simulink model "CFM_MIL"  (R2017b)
settings: Solver=FixedStepDiscrete  StartTime=0.0  StopTime=10.0  FixedStep=0.01  RelTol=1e-3  EnableMultiTasking=on
undefined symbols (not defined in the file): ASWTYPE_FALSE, CFM_CONST0_NUMB, CFM_CONST14_NUMB, CFM_CONST1_NUMB, CFM_CONST6_NUMB, CFM_CONST8_NUMB, Enum_CFMBusBarCell, Enum_CFMNTCTemp
libraries: AIWAYS_Powertrain_BMS_lib x17

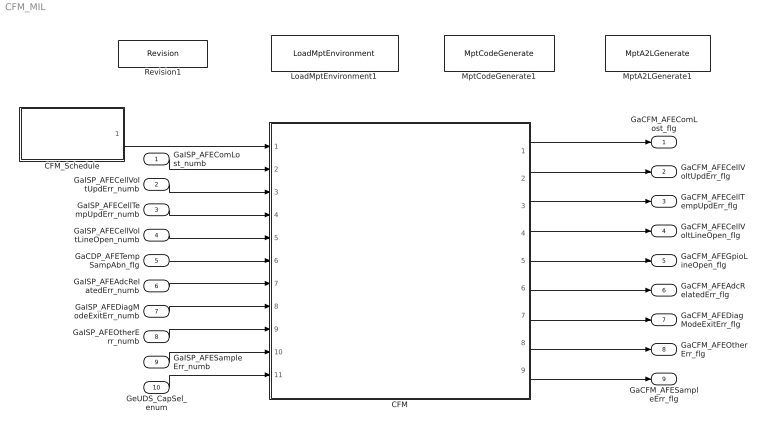
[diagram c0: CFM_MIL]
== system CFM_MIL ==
  GaISP_AFEComLost_numb : Inport
  GaISP_AFECellVoltUpdErr_numb : Inport  Port=2
  GaISP_AFECellTempUpdErr_numb : Inport  Port=3
  GaISP_AFECellVoltLineOpen_numb : Inport  Port=4
  GaCDP_AFETempSampAbn_flg : Inport  Port=5
  GaISP_AFEAdcRelatedErr_numb : Inport  Port=6
  GaISP_AFEDiagModeExitErr_numb : Inport  Port=7
  GaISP_AFEOtherErr_numb : Inport  Port=8
  GaISP_AFESampleErr_numb : Inport  Port=9
  GeUDS_CapSel_enum : Inport  Port=10
  CFM : Subsystem
  CFM_Schedule : Stateflow chart  TreatAsAtomicUnit=on
  LoadMptEnvironment1 : AIWAYS_Powertrain_BMS_lib/Config/LoadMptEnvironment  ProjectName=Comm  SuppierID=NewPlatformUAES
  MptA2LGenerate1 : AIWAYS_Powertrain_BMS_lib/Config/MptA2LGenerate  SystemSampleTime=-1
  MptCodeGenerate1 : AIWAYS_Powertrain_BMS_lib/Config/MptCodeGenerate  SystemSampleTime=-1
  Revision1 : AIWAYS_Powertrain_BMS_lib/Config/Revision  curVersion='M103C102'  newVersion='M103C102'
  GaCFM_AFEComLost_flg : Outport
  GaCFM_AFECellVoltUpdErr_flg : Outport  Port=2
  GaCFM_AFECellTempUpdErr_flg : Outport  Port=3
  GaCFM_AFECellVoltLineOpen_flg : Outport  Port=4
  GaCFM_AFEGpioLineOpen_flg : Outport  Port=5
  GaCFM_AFEAdcRelatedErr_flg : Outport  Port=6
  GaCFM_AFEDiagModeExitErr_flg : Outport  Port=7
  GaCFM_AFEOtherErr_flg : Outport  Port=8
  GaCFM_AFESampleErr_flg : Outport  Port=9
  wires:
  GaISP_AFEComLost_numb/1 -> CFM/2(GaISP_AFEComLost_numb)
  GaISP_AFECellVoltUpdErr_numb/1 -> CFM/3(GaISP_AFECellVoltUpdErr_numb)
  GaISP_AFECellTempUpdErr_numb/1 -> CFM/4(GaISP_AFECellTempUpdErr_numb)
  GaISP_AFECellVoltLineOpen_numb/1 -> CFM/5(GaISP_AFECellVoltLineOpen_numb)
  GaCDP_AFETempSampAbn_flg/1 -> CFM/6(GaCDP_AFETempSampAbn_flg)
  GaISP_AFEAdcRelatedErr_numb/1 -> CFM/7(GaISP_AFEAdcRelatedErr_numb)
  GaISP_AFEDiagModeExitErr_numb/1 -> CFM/8(GaISP_AFEDiagModeExitErr_numb)
  GaISP_AFEOtherErr_numb/1 -> CFM/9(GaISP_AFEOtherErr_numb)
  GaISP_AFESampleErr_numb/1 -> CFM/10(GaISP_AFESampleErr_numb)
  CFM_Schedule/1(CFM_CMCFltMag_20ms()) -> CFM/1(CFM_CMCFltMag_20ms)
  CFM/1(GaCFM_AFEComLost_flg) -> GaCFM_AFEComLost_flg/1
  CFM/2(GaCFM_AFECellVoltUpdErr_flg) -> GaCFM_AFECellVoltUpdErr_flg/1
  CFM/3(GaCFM_AFECellTempUpdErr_flg) -> GaCFM_AFECellTempUpdErr_flg/1
  CFM/4(GaCFM_AFECellVoltLineOpen_flg) -> GaCFM_AFECellVoltLineOpen_flg/1
  CFM/5(GaCFM_AFEGpioLineOpen_flg) -> GaCFM_AFEGpioLineOpen_flg/1
  CFM/6(GaCFM_AFEAdcRelatedErr_flg) -> GaCFM_AFEAdcRelatedErr_flg/1
  CFM/7(GaCFM_AFEDiagModeExitErr_flg) -> GaCFM_AFEDiagModeExitErr_flg/1
  CFM/8(GaCFM_AFEOtherErr_flg) -> GaCFM_AFEOtherErr_flg/1
  CFM/9(GaCFM_AFESampleErr_flg) -> GaCFM_AFESampleErr_flg/1
  GeUDS_CapSel_enum/1 -> CFM/11(GeUDS_CapSel_enum)

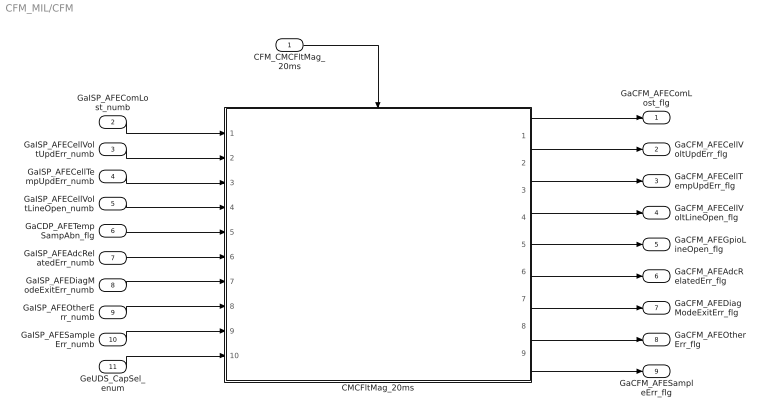
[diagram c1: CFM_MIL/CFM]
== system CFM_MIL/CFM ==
  CFM_CMCFltMag_20ms : Inport
  GaISP_AFEComLost_numb : Inport  Port=2
  GaISP_AFECellVoltUpdErr_numb : Inport  Port=3
  GaISP_AFECellTempUpdErr_numb : Inport  Port=4
  GaISP_AFECellVoltLineOpen_numb : Inport  Port=5
  GaCDP_AFETempSampAbn_flg : Inport  Port=6
  GaISP_AFEAdcRelatedErr_numb : Inport  Port=7
  GaISP_AFEDiagModeExitErr_numb : Inport  Port=8
  GaISP_AFEOtherErr_numb : Inport  Port=9
  GaISP_AFESampleErr_numb : Inport  Port=10
  GeUDS_CapSel_enum : Inport  Port=11
  CMCFltMag_20ms : Subsystem
  GaCFM_AFEComLost_flg : Outport
  GaCFM_AFECellVoltUpdErr_flg : Outport  Port=2
  GaCFM_AFECellTempUpdErr_flg : Outport  Port=3
  GaCFM_AFECellVoltLineOpen_flg : Outport  Port=4
  GaCFM_AFEGpioLineOpen_flg : Outport  Port=5
  GaCFM_AFEAdcRelatedErr_flg : Outport  Port=6
  GaCFM_AFEDiagModeExitErr_flg : Outport  Port=7
  GaCFM_AFEOtherErr_flg : Outport  Port=8
  GaCFM_AFESampleErr_flg : Outport  Port=9
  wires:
  CFM_CMCFltMag_20ms/1 -> CMCFltMag_20ms/Trigger
  GaISP_AFEComLost_numb/1 -> CMCFltMag_20ms/1(GaISP_AFEComLost_numb)
  GaISP_AFECellVoltUpdErr_numb/1 -> CMCFltMag_20ms/2(GaISP_AFECellVoltUpdErr_numb)
  GaISP_AFECellTempUpdErr_numb/1 -> CMCFltMag_20ms/3(GaISP_AFECellTempUpdErr_numb)
  GaISP_AFECellVoltLineOpen_numb/1 -> CMCFltMag_20ms/4(GaISP_AFECellVoltLineOpen_numb)
  GaCDP_AFETempSampAbn_flg/1 -> CMCFltMag_20ms/5(GaCDP_AFETempSampAbn_flg)
  GaISP_AFEAdcRelatedErr_numb/1 -> CMCFltMag_20ms/6(GaISP_AFEAdcRelatedErr_numb)
  GaISP_AFEDiagModeExitErr_numb/1 -> CMCFltMag_20ms/7(GaISP_AFEDiagModeExitErr_numb)
  GaISP_AFEOtherErr_numb/1 -> CMCFltMag_20ms/8(GaISP_AFEOtherErr_numb)
  GaISP_AFESampleErr_numb/1 -> CMCFltMag_20ms/9(GaISP_AFESampleErr_numb)
  CMCFltMag_20ms/1(GaCFM_AFEComLost_flg) -> GaCFM_AFEComLost_flg/1
  CMCFltMag_20ms/2(GaCFM_AFECellVoltUpdErr_flg) -> GaCFM_AFECellVoltUpdErr_flg/1
  CMCFltMag_20ms/3(GaCFM_AFECellTempUpdErr_flg) -> GaCFM_AFECellTempUpdErr_flg/1
  CMCFltMag_20ms/4(GaCFM_AFECellVoltLineOpen_flg) -> GaCFM_AFECellVoltLineOpen_flg/1
  CMCFltMag_20ms/5(GaCFM_AFEGpioLineOpen_flg) -> GaCFM_AFEGpioLineOpen_flg/1
  CMCFltMag_20ms/6(GaCFM_AFEAdcRelatedErr_flg) -> GaCFM_AFEAdcRelatedErr_flg/1
  CMCFltMag_20ms/7(GaCFM_AFEDiagModeExitErr_flg) -> GaCFM_AFEDiagModeExitErr_flg/1
  CMCFltMag_20ms/8(GaCFM_AFEOtherErr_flg) -> GaCFM_AFEOtherErr_flg/1
  CMCFltMag_20ms/9(GaCFM_AFESampleErr_flg) -> GaCFM_AFESampleErr_flg/1
  GeUDS_CapSel_enum/1 -> CMCFltMag_20ms/10(GeUDS_CapSel_enum)

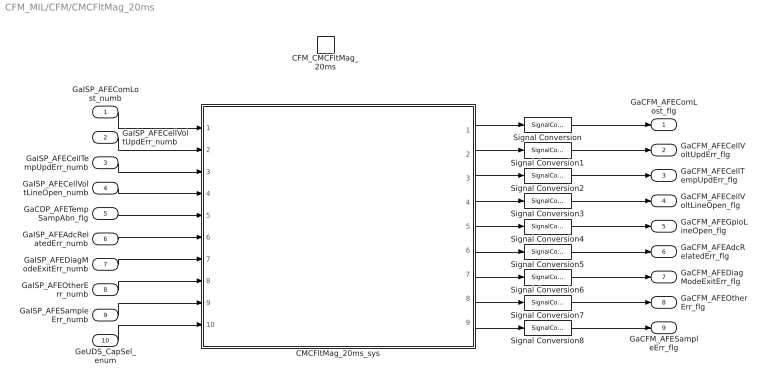
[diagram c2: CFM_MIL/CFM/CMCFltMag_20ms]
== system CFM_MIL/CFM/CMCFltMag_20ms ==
  GaISP_AFEComLost_numb : Inport
  GaISP_AFECellVoltUpdErr_numb : Inport  Port=2
  GaISP_AFECellTempUpdErr_numb : Inport  Port=3
  GaISP_AFECellVoltLineOpen_numb : Inport  Port=4
  GaCDP_AFETempSampAbn_flg : Inport  Port=5
  GaISP_AFEAdcRelatedErr_numb : Inport  Port=6
  GaISP_AFEDiagModeExitErr_numb : Inport  Port=7
  GaISP_AFEOtherErr_numb : Inport  Port=8
  GaISP_AFESampleErr_numb : Inport  Port=9
  GeUDS_CapSel_enum : Inport  Port=10
  CFM_CMCFltMag_20ms : TriggerPort  TriggerType=function-call  VariantControl=(inherit)
  CMCFltMag_20ms_sys : Subsystem
  Signal Conversion{,1..8} (9 alike) : SignalConversion  ConversionOutput=Contiguous copy  OverrideOpt=off
  GaCFM_AFEComLost_flg : Outport
  GaCFM_AFECellVoltUpdErr_flg : Outport  Port=2
  GaCFM_AFECellTempUpdErr_flg : Outport  Port=3
  GaCFM_AFECellVoltLineOpen_flg : Outport  Port=4
  GaCFM_AFEGpioLineOpen_flg : Outport  Port=5
  GaCFM_AFEAdcRelatedErr_flg : Outport  Port=6
  GaCFM_AFEDiagModeExitErr_flg : Outport  Port=7
  GaCFM_AFEOtherErr_flg : Outport  Port=8
  GaCFM_AFESampleErr_flg : Outport  Port=9
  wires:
  GaISP_AFEComLost_numb/1 -> CMCFltMag_20ms_sys/1(GaISP_AFEComLost_numb)
  GaISP_AFECellVoltUpdErr_numb/1 -> CMCFltMag_20ms_sys/2(GaISP_AFECellVoltUpdErr_numb)
  GaISP_AFECellTempUpdErr_numb/1 -> CMCFltMag_20ms_sys/3(GaISP_AFECellTempUpdErr_numb)
  GaISP_AFECellVoltLineOpen_numb/1 -> CMCFltMag_20ms_sys/4(GaISP_AFECellVoltLineOpen_numb)
  GaCDP_AFETempSampAbn_flg/1 -> CMCFltMag_20ms_sys/5(GaCDP_AFETempSampAbn_flg)
  GaISP_AFEAdcRelatedErr_numb/1 -> CMCFltMag_20ms_sys/6(GaISP_AFEAdcRelatedErr_numb)
  GaISP_AFEDiagModeExitErr_numb/1 -> CMCFltMag_20ms_sys/7(GaISP_AFEDiagModeExitErr_numb)
  GaISP_AFEOtherErr_numb/1 -> CMCFltMag_20ms_sys/8(GaISP_AFEOtherErr_numb)
  GaISP_AFESampleErr_numb/1 -> CMCFltMag_20ms_sys/9(GaISP_AFESampleErr_numb)
  CMCFltMag_20ms_sys/1(GaCFM_AFEComLost_flg) -> Signal Conversion/1
  CMCFltMag_20ms_sys/2(GaCFM_AFECellVoltUpdErr_flg) -> Signal Conversion1/1
  CMCFltMag_20ms_sys/3(GaCFM_AFECellTempUpdErr_flg) -> Signal Conversion2/1
  CMCFltMag_20ms_sys/4(GaCFM_AFECellVoltLineOpen_flg) -> Signal Conversion3/1
  CMCFltMag_20ms_sys/5(GaCFM_AFEGpioLineOpen_flg) -> Signal Conversion4/1
  CMCFltMag_20ms_sys/6(GaCFM_AFEAdcRelatedErr_flg) -> Signal Conversion5/1
  CMCFltMag_20ms_sys/7(GaCFM_AFEDiagModeExitErr_flg) -> Signal Conversion6/1
  CMCFltMag_20ms_sys/8(GaCFM_AFEOtherErr_flg) -> Signal Conversion7/1
  CMCFltMag_20ms_sys/9(GaCFM_AFESampleErr_flg) -> Signal Conversion8/1
  Signal Conversion/1 -> GaCFM_AFEComLost_flg/1
  Signal Conversion1/1 -> GaCFM_AFECellVoltUpdErr_flg/1
  Signal Conversion2/1 -> GaCFM_AFECellTempUpdErr_flg/1
  Signal Conversion3/1 -> GaCFM_AFECellVoltLineOpen_flg/1
  Signal Conversion4/1 -> GaCFM_AFEGpioLineOpen_flg/1
  Signal Conversion5/1 -> GaCFM_AFEAdcRelatedErr_flg/1
  Signal Conversion6/1 -> GaCFM_AFEDiagModeExitErr_flg/1
  Signal Conversion7/1 -> GaCFM_AFEOtherErr_flg/1
  Signal Conversion8/1 -> GaCFM_AFESampleErr_flg/1
  GeUDS_CapSel_enum/1 -> CMCFltMag_20ms_sys/10(GeUDS_CapSel_enum)

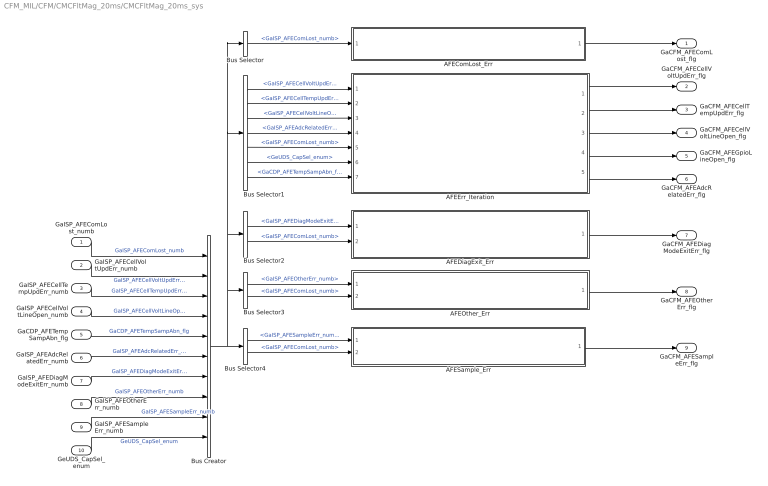
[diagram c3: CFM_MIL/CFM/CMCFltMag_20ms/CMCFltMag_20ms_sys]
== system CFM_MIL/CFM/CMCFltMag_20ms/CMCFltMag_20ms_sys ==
  GaISP_AFEComLost_numb : Inport
  GaISP_AFECellVoltUpdErr_numb : Inport  Port=2
  GaISP_AFECellTempUpdErr_numb : Inport  Port=3
  GaISP_AFECellVoltLineOpen_numb : Inport  Port=4
  GaCDP_AFETempSampAbn_flg : Inport  Port=5
  GaISP_AFEAdcRelatedErr_numb : Inport  Port=6
  GaISP_AFEDiagModeExitErr_numb : Inport  Port=7
  GaISP_AFEOtherErr_numb : Inport  Port=8
  GaISP_AFESampleErr_numb : Inport  Port=9
  GeUDS_CapSel_enum : Inport  Port=10
  AFEComLost_Err : Subsystem
  AFEDiagExit_Err : Subsystem
  AFEErr_Iteration : Subsystem
  AFEOther_Err : Subsystem
  AFESample_Err : Subsystem
  Bus Creator : BusCreator  Inputs=10
  Bus Selector : BusSelector  OutputSignals=GaISP_AFEComLost_numb
  Bus Selector1 : BusSelector  OutputSignals=GaISP_AFECellVoltUpdErr_numb,GaISP_AFECellTempUpdErr_numb,GaISP_AFECellVoltLineOpen_numb,GaISP_AFEAdcRelatedErr_numb,GaISP_AFEComLost_numb,GeUDS_CapSel_enum,GaCDP_AFETempSampAbn_flg
  Bus Selector2 : BusSelector  OutputSignals=GaISP_AFEDiagModeExitErr_numb,GaISP_AFEComLost_numb
  Bus Selector3 : BusSelector  OutputSignals=GaISP_AFEOtherErr_numb,GaISP_AFEComLost_numb
  Bus Selector4 : BusSelector  OutputSignals=GaISP_AFESampleErr_numb,GaISP_AFEComLost_numb
  GaCFM_AFEComLost_flg : Outport
  GaCFM_AFECellVoltUpdErr_flg : Outport  Port=2
  GaCFM_AFECellTempUpdErr_flg : Outport  Port=3
  GaCFM_AFECellVoltLineOpen_flg : Outport  Port=4
  GaCFM_AFEGpioLineOpen_flg : Outport  Port=5
  GaCFM_AFEAdcRelatedErr_flg : Outport  Port=6
  GaCFM_AFEDiagModeExitErr_flg : Outport  Port=7
  GaCFM_AFEOtherErr_flg : Outport  Port=8
  GaCFM_AFESampleErr_flg : Outport  Port=9
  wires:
  AFEComLost_Err/1(GaCFM_AFEComLost_flg) -> GaCFM_AFEComLost_flg/1
  AFEDiagExit_Err/1(GaCFM_AFEDiagModeExitErr_flg) -> GaCFM_AFEDiagModeExitErr_flg/1
  AFEOther_Err/1(GaCFM_AFEOtherErr_flg) -> GaCFM_AFEOtherErr_flg/1
  AFESample_Err/1(GaCFM_AFESampleErr_flg) -> GaCFM_AFESampleErr_flg/1
  AFEErr_Iteration/1(GaCFM_AFECellVoltUpdErr_flg) -> GaCFM_AFECellVoltUpdErr_flg/1
  AFEErr_Iteration/2(GaCFM_AFECellTempUpdErr_flg) -> GaCFM_AFECellTempUpdErr_flg/1
  AFEErr_Iteration/3(GaCFM_AFECellVoltLineOpen_flg) -> GaCFM_AFECellVoltLineOpen_flg/1
  AFEErr_Iteration/4(GaCFM_AFEGpioLineOpen_flg) -> GaCFM_AFEGpioLineOpen_flg/1
  AFEErr_Iteration/5(GaCFM_AFEAdcRelatedErr_flg) -> GaCFM_AFEAdcRelatedErr_flg/1
  GaISP_AFEComLost_numb/1 -> Bus Creator/1  "GaISP_AFEComLost_numb"
  GaISP_AFECellVoltUpdErr_numb/1 -> Bus Creator/2  "GaISP_AFECellVoltUpdErr_numb"
  GaISP_AFECellTempUpdErr_numb/1 -> Bus Creator/3  "GaISP_AFECellTempUpdErr_numb"
  GaISP_AFECellVoltLineOpen_numb/1 -> Bus Creator/4  "GaISP_AFECellVoltLineOpen_numb"
  GaCDP_AFETempSampAbn_flg/1 -> Bus Creator/5  "GaCDP_AFETempSampAbn_flg"
  GaISP_AFEAdcRelatedErr_numb/1 -> Bus Creator/6  "GaISP_AFEAdcRelatedErr_numb"
  GaISP_AFEDiagModeExitErr_numb/1 -> Bus Creator/7  "GaISP_AFEDiagModeExitErr_numb"
  GaISP_AFEOtherErr_numb/1 -> Bus Creator/8  "GaISP_AFEOtherErr_numb"
  GaISP_AFESampleErr_numb/1 -> Bus Creator/9  "GaISP_AFESampleErr_numb"
  Bus Creator/1 -> Bus Selector/1, Bus Selector1/1, Bus Selector2/1, Bus Selector3/1, Bus Selector4/1
  Bus Selector/1 -> AFEComLost_Err/1(GaISP_AFEComLost_numb)  "<GaISP_AFEComLost_numb>"
  Bus Selector2/1 -> AFEDiagExit_Err/1(GaISP_AFEDiagModeExitErr_numb)  "<GaISP_AFEDiagModeExitErr_numb>"
  Bus Selector2/2 -> AFEDiagExit_Err/2(GaISP_AFEComLost_numb)  "<GaISP_AFEComLost_numb>"
  Bus Selector3/1 -> AFEOther_Err/1(GaISP_AFEOtherErr_numb)  "<GaISP_AFEOtherErr_numb>"
  Bus Selector3/2 -> AFEOther_Err/2(GaISP_AFEComLost_numb)  "<GaISP_AFEComLost_numb>"
  Bus Selector4/2 -> AFESample_Err/2(GaISP_AFEComLost_numb)  "<GaISP_AFEComLost_numb>"
  Bus Selector4/1 -> AFESample_Err/1(GaISP_AFESampleErr_numb)  "<GaISP_AFESampleErr_numb>"
  GeUDS_CapSel_enum/1 -> Bus Creator/10  "GeUDS_CapSel_enum"
  Bus Selector1/1 -> AFEErr_Iteration/1(GaISP_AFECellVoltUpdErr_numb)  "<GaISP_AFECellVoltUpdErr_numb>"
  Bus Selector1/2 -> AFEErr_Iteration/2(GaISP_AFECellTempUpdErr_numb)  "<GaISP_AFECellTempUpdErr_numb>"
  Bus Selector1/3 -> AFEErr_Iteration/3(GaISP_AFECellVoltLineOpen_numb)  "<GaISP_AFECellVoltLineOpen_numb>"
  Bus Selector1/4 -> AFEErr_Iteration/4(GaISP_AFEAdcRelatedErr_numb)  "<GaISP_AFEAdcRelatedErr_numb>"
  Bus Selector1/5 -> AFEErr_Iteration/5(GaISP_AFEComLost_numb)  "<GaISP_AFEComLost_numb>"
  Bus Selector1/6 -> AFEErr_Iteration/6(GeUDS_CapSel_enum)  "<GeUDS_CapSel_enum>"
  Bus Selector1/7 -> AFEErr_Iteration/7(GaCDP_AFETempSampAbn_flg)  "<GaCDP_AFETempSampAbn_flg>"

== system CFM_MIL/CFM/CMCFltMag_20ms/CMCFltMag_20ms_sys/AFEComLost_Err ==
  GaISP_AFEComLost_numb : Inport
  CFM_GaCFM_AFEComLost_flg : AIWAYS_Powertrain_BMS_lib/Signals/OverWrite  OverWrite_Value=CaCFM_AFEComLostOvr_flg  OverWrite_flag=CbCFM_AFEComLostOvrSwt_flg
  Constant3 : Constant  Value=CFM_CONST0_NUMB
  Relational Operator2 : RelationalOperator  Operator=~=  OutDataTypeStr=boolean
  GaCFM_AFEComLost_flg : Outport
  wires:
  GaISP_AFEComLost_numb/1 -> Relational Operator2/1
  Constant3/1 -> Relational Operator2/2
  CFM_GaCFM_AFEComLost_flg/1 -> GaCFM_AFEComLost_flg/1  "GaCFM_AFEComLost_flg"
  Relational Operator2/1 -> CFM_GaCFM_AFEComLost_flg/1  "LaCFM_AFEComLost_flg"

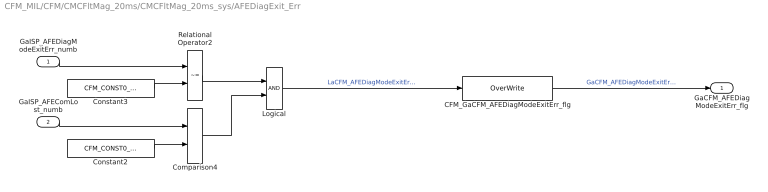
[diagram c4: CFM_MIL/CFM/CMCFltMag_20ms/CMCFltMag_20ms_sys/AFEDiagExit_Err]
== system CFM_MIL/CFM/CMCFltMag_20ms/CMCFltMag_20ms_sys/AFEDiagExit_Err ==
  GaISP_AFEDiagModeExitErr_numb : Inport
  GaISP_AFEComLost_numb : Inport  Port=2
  CFM_GaCFM_AFEDiagModeExitErr_flg : AIWAYS_Powertrain_BMS_lib/Signals/OverWrite  OverWrite_Value=CaCFM_AFEDiagModeExitErrOvr_flg  OverWrite_flag=CbCFM_AFEDiagModeExitErrOvrSwt_flg
  Comparison4 : RelationalOperator  Operator===  OutDataTypeStr=boolean
  Constant2 : Constant  Value=CFM_CONST0_NUMB
  Constant3 : Constant  Value=CFM_CONST0_NUMB
  Logical : Logic  OutDataTypeStr=boolean
  Relational Operator2 : RelationalOperator  Operator=~=  OutDataTypeStr=boolean
  GaCFM_AFEDiagModeExitErr_flg : Outport
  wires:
  Constant3/1 -> Relational Operator2/2
  GaISP_AFEDiagModeExitErr_numb/1 -> Relational Operator2/1
  CFM_GaCFM_AFEDiagModeExitErr_flg/1 -> GaCFM_AFEDiagModeExitErr_flg/1  "GaCFM_AFEDiagModeExitErr_flg"
  Constant2/1 -> Comparison4/2
  GaISP_AFEComLost_numb/1 -> Comparison4/1
  Relational Operator2/1 -> Logical/1
  Comparison4/1 -> Logical/2
  Logical/1 -> CFM_GaCFM_AFEDiagModeExitErr_flg/1  "LaCFM_AFEDiagModeExitErr_flg"

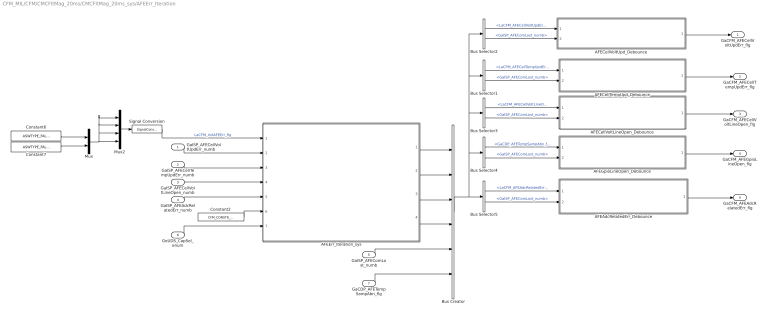
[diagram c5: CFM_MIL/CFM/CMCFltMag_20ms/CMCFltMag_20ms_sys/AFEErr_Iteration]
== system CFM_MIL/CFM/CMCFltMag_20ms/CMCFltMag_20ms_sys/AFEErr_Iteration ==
  GaISP_AFECellVoltUpdErr_numb : Inport
  GaISP_AFECellTempUpdErr_numb : Inport  Port=2
  GaISP_AFECellVoltLineOpen_numb : Inport  Port=3
  GaISP_AFEAdcRelatedErr_numb : Inport  Port=4
  GaISP_AFEComLost_numb : Inport  Port=5
  GeUDS_CapSel_enum : Inport  Port=6
  GaCDP_AFETempSampAbn_flg : Inport  Port=7
  AFEAdcRelatedErr_Debounce : Subsystem
  AFECellTempUpd_Debounce : Subsystem
  AFECellVoltLineOpen_Debounce : Subsystem
  AFECellVoltUpd_Debounce : Subsystem
  AFEErr_Iteration_sys : Subsystem
  AFEGpioLineOpen_Debounce : Subsystem
  Bus Creator : BusCreator  Inputs=6
  Bus Selector1 : BusSelector  OutputSignals=LaCFM_AFECellTempUpdErr_flg,GaISP_AFEComLost_numb
  Bus Selector2 : BusSelector  OutputSignals=LaCFM_AFECellVoltUpdErr_flg,GaISP_AFEComLost_numb
  Bus Selector3 : BusSelector  OutputSignals=LaCFM_AFECellVoltLineOpen_flg,GaISP_AFEComLost_numb
  Bus Selector4 : BusSelector  OutputSignals=GaCDP_AFETempSampAbn_flg,GaISP_AFEComLost_numb
  Bus Selector5 : BusSelector  OutputSignals=LaCFM_AFEAdcRelatedErr_flg,GaISP_AFEComLost_numb
  Constant2 : Constant  Value=CFM_CONST8_NUMB
  Constant6 : Constant  Value=ASWTYPE_FALSE
  Constant7 : Constant  Value=ASWTYPE_FALSE
  Mux : Mux  Inputs=2
  Mux2 : Mux
  Signal Conversion : SignalConversion  ConversionOutput=Contiguous copy  OverrideOpt=off
  GaCFM_AFECellVoltUpdErr_flg : Outport
  GaCFM_AFECellTempUpdErr_flg : Outport  Port=2
  GaCFM_AFECellVoltLineOpen_flg : Outport  Port=3
  GaCFM_AFEGpioLineOpen_flg : Outport  Port=4
  GaCFM_AFEAdcRelatedErr_flg : Outport  Port=5
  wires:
  GaISP_AFECellTempUpdErr_numb/1 -> AFEErr_Iteration_sys/3(GaISP_AFECellTempUpdErr_numb)
  Signal Conversion/1 -> AFEErr_Iteration_sys/1(LaCFM_InitAFEErr_flg)  "LaCFM_InitAFEErr_flg"
  GaISP_AFECellVoltLineOpen_numb/1 -> AFEErr_Iteration_sys/4(GaISP_AFECellVoltLineOpen_numb)
  Constant2/1 -> AFEErr_Iteration_sys/6(CFM_CONST8_NUMB)
  GaISP_AFECellVoltUpdErr_numb/1 -> AFEErr_Iteration_sys/2(GaISP_AFECellVoltUpdErr_numb)
  GaISP_AFEAdcRelatedErr_numb/1 -> AFEErr_Iteration_sys/5(GaISP_AFEAdcRelatedErr_numb)
  Constant6/1 -> Mux/1
  Mux2/1 -> Signal Conversion/1
  Mux/1 -> Mux2/1, Mux2/2, Mux2/3, Mux2/4
  Constant7/1 -> Mux/2
  AFECellVoltUpd_Debounce/1(GaCFM_AFECellVoltUpdErr_flg) -> GaCFM_AFECellVoltUpdErr_flg/1
  AFECellTempUpd_Debounce/1(GaCFM_AFECellTempUpdErr_flg) -> GaCFM_AFECellTempUpdErr_flg/1
  AFECellVoltLineOpen_Debounce/1(GaCFM_AFECellVoltLineOpen_flg) -> GaCFM_AFECellVoltLineOpen_flg/1
  AFEGpioLineOpen_Debounce/1(GaCFM_AFEGpioLineOpen_flg) -> GaCFM_AFEGpioLineOpen_flg/1
  AFEAdcRelatedErr_Debounce/1(GaCFM_AFEAdcRelatedErr_flg) -> GaCFM_AFEAdcRelatedErr_flg/1
  AFEErr_Iteration_sys/1(LaCFM_AFECellVoltUpdErr_flg) -> Bus Creator/1
  AFEErr_Iteration_sys/2(LaCFM_AFECellTempUpdErr_flg) -> Bus Creator/2
  AFEErr_Iteration_sys/3(LaCFM_AFECellVoltLineOpen_flg) -> Bus Creator/3
  AFEErr_Iteration_sys/4(LaCFM_AFEAdcRelatedErr_flg) -> Bus Creator/4
  GaISP_AFEComLost_numb/1 -> Bus Creator/5
  Bus Creator/1 -> Bus Selector1/1, Bus Selector2/1, Bus Selector3/1, Bus Selector4/1, Bus Selector5/1
  Bus Selector2/1 -> AFECellVoltUpd_Debounce/1(LaCFM_AFECellVoltUpdErr_flg)  "<LaCFM_AFECellVoltUpdErr_flg>"
  Bus Selector2/2 -> AFECellVoltUpd_Debounce/2(GaISP_AFEComLost_numb)  "<GaISP_AFEComLost_numb>"
  Bus Selector1/1 -> AFECellTempUpd_Debounce/1(LaCFM_AFECellTempUpdErr_flg)  "<LaCFM_AFECellTempUpdErr_flg>"
  Bus Selector1/2 -> AFECellTempUpd_Debounce/2(GaISP_AFEComLost_numb)  "<GaISP_AFEComLost_numb>"
  Bus Selector3/1 -> AFECellVoltLineOpen_Debounce/1(LaCFM_AFECellVoltLineOpen_flg)  "<LaCFM_AFECellVoltLineOpen_flg>"
  Bus Selector3/2 -> AFECellVoltLineOpen_Debounce/2(GaISP_AFEComLost_numb)  "<GaISP_AFEComLost_numb>"
  Bus Selector4/1 -> AFEGpioLineOpen_Debounce/1(GaCDP_AFETempSampAbn_flg)  "<GaCDP_AFETempSampAbn_flg>"
  Bus Selector4/2 -> AFEGpioLineOpen_Debounce/2(GaISP_AFEComLost_numb)  "<GaISP_AFEComLost_numb>"
  Bus Selector5/1 -> AFEAdcRelatedErr_Debounce/1(LaCFM_AFEAdcRelatedErr_flg)  "<LaCFM_AFEAdcRelatedErr_flg>"
  Bus Selector5/2 -> AFEAdcRelatedErr_Debounce/2(GaISP_AFEComLost_numb)  "<GaISP_AFEComLost_numb>"
  GeUDS_CapSel_enum/1 -> AFEErr_Iteration_sys/7(GeUDS_CapSel_enum)
  GaCDP_AFETempSampAbn_flg/1 -> Bus Creator/6

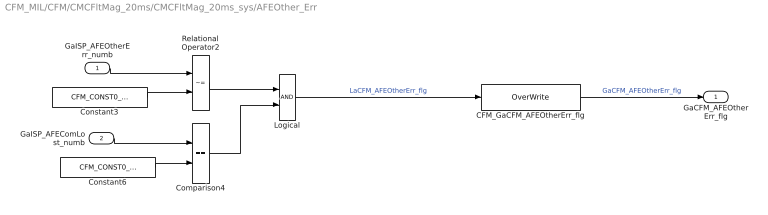
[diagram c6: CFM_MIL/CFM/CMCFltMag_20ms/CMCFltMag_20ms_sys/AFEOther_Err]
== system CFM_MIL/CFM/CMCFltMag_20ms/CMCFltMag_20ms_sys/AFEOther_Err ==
  GaISP_AFEOtherErr_numb : Inport
  GaISP_AFEComLost_numb : Inport  Port=2
  CFM_GaCFM_AFEOtherErr_flg : AIWAYS_Powertrain_BMS_lib/Signals/OverWrite  OverWrite_Value=CaCFM_AFEOtherErrOvr_flg  OverWrite_flag=CbCFM_AFEOtherErrOvrSwt_flg
  Comparison4 : RelationalOperator  Operator===  OutDataTypeStr=boolean
  Constant3 : Constant  Value=CFM_CONST0_NUMB
  Constant6 : Constant  Value=CFM_CONST0_NUMB
  Logical : Logic  OutDataTypeStr=boolean
  Relational Operator2 : RelationalOperator  Operator=~=  OutDataTypeStr=boolean
  GaCFM_AFEOtherErr_flg : Outport
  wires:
  GaISP_AFEOtherErr_numb/1 -> Relational Operator2/1
  Constant3/1 -> Relational Operator2/2
  CFM_GaCFM_AFEOtherErr_flg/1 -> GaCFM_AFEOtherErr_flg/1  "GaCFM_AFEOtherErr_flg"
  Relational Operator2/1 -> Logical/1
  Constant6/1 -> Comparison4/2
  GaISP_AFEComLost_numb/1 -> Comparison4/1
  Comparison4/1 -> Logical/2
  Logical/1 -> CFM_GaCFM_AFEOtherErr_flg/1  "LaCFM_AFEOtherErr_flg"

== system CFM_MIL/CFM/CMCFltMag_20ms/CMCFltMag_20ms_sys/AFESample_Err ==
  GaISP_AFESampleErr_numb : Inport
  GaISP_AFEComLost_numb : Inport  Port=2
  CFM_GaCFM_AFESampleErr_flg : AIWAYS_Powertrain_BMS_lib/Signals/OverWrite  OverWrite_Value=CaCFM_AFESampleErrOvr_flg  OverWrite_flag=CbCFM_AFESampleErrOvrSwt_flg
  Constant2 : Constant  Value=CFM_CONST0_NUMB
  Constant3 : Constant  Value=CFM_CONST0_NUMB
  Logical : Logic  OutDataTypeStr=boolean
  Relational Operator1 : RelationalOperator  Operator===  OutDataTypeStr=boolean
  Relational Operator2 : RelationalOperator  Operator=~=  OutDataTypeStr=boolean
  GaCFM_AFESampleErr_flg : Outport
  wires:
  GaISP_AFESampleErr_numb/1 -> Relational Operator2/1
  Constant3/1 -> Relational Operator2/2
  CFM_GaCFM_AFESampleErr_flg/1 -> GaCFM_AFESampleErr_flg/1  "GaCFM_AFESampleErr_flg"
  Logical/1 -> CFM_GaCFM_AFESampleErr_flg/1  "LaCFM_AFESampleErr_flg"
  Constant2/1 -> Relational Operator1/2
  GaISP_AFEComLost_numb/1 -> Relational Operator1/1
  Relational Operator2/1 -> Logical/1
  Relational Operator1/1 -> Logical/2

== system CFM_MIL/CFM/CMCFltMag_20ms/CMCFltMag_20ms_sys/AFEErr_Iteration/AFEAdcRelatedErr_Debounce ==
  LaCFM_AFEAdcRelatedErr_flg : Inport
  GaISP_AFEComLost_numb : Inport  Port=2
  CFM_GaCFM_AFEAdcRelatedErr_flg : AIWAYS_Powertrain_BMS_lib/Signals/OverWrite  OverWrite_Value=CaCFM_AFEAdcRelatedErrOvr_flg  OverWrite_flag=CbCFM_AFEAdcRelatedErrOvrSwt_flg
  Comparison4 : RelationalOperator  Operator===  OutDataTypeStr=boolean
  Constant3 : Constant  Value=CFM_CONST0_NUMB
  Logical : Logic  OutDataTypeStr=boolean
  GaCFM_AFEAdcRelatedErr_flg : Outport
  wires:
  LaCFM_AFEAdcRelatedErr_flg/1 -> Logical/1
  CFM_GaCFM_AFEAdcRelatedErr_flg/1 -> GaCFM_AFEAdcRelatedErr_flg/1  "GaCFM_AFEAdcRelatedErr_flg"
  Logical/1 -> CFM_GaCFM_AFEAdcRelatedErr_flg/1
  GaISP_AFEComLost_numb/1 -> Comparison4/1
  Comparison4/1 -> Logical/2
  Constant3/1 -> Comparison4/2

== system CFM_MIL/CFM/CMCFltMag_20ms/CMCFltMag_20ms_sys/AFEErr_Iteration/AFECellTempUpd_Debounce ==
  LaCFM_AFECellTempUpdErr_flg : Inport
  GaISP_AFEComLost_numb : Inport  Port=2
  CFM_GaCFM_AFECellTempUpdErr_flg : AIWAYS_Powertrain_BMS_lib/Signals/OverWrite  OverWrite_Value=CaCFM_AFECellTempUpdErrOvr_flg  OverWrite_flag=CbCFM_AFECellTempUpdErrOvrSwt_flg
  Comparison4 : RelationalOperator  Operator===  OutDataTypeStr=boolean
  Constant3 : Constant  Value=CFM_CONST0_NUMB
  Logical : Logic  OutDataTypeStr=boolean
  GaCFM_AFECellTempUpdErr_flg : Outport
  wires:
  CFM_GaCFM_AFECellTempUpdErr_flg/1 -> GaCFM_AFECellTempUpdErr_flg/1  "GaCFM_AFECellTempUpdErr_flg"
  Logical/1 -> CFM_GaCFM_AFECellTempUpdErr_flg/1
  GaISP_AFEComLost_numb/1 -> Comparison4/1
  Comparison4/1 -> Logical/2
  LaCFM_AFECellTempUpdErr_flg/1 -> Logical/1
  Constant3/1 -> Comparison4/2

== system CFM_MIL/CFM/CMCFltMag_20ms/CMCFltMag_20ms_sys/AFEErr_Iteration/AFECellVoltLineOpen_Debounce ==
  LaCFM_AFECellVoltLineOpen_flg : Inport
  GaISP_AFEComLost_numb : Inport  Port=2
  CFM_GaCFM_AFECellVoltLineOpen_flg : AIWAYS_Powertrain_BMS_lib/Signals/OverWrite  OverWrite_Value=CaCFM_AFECellVoltLineOpenOvr_flg  OverWrite_flag=CbCFM_AFECellVoltLineOpenOvrSwt_flg
  Comparison4 : RelationalOperator  Operator===  OutDataTypeStr=boolean
  Constant2 : Constant  Value=CFM_CONST0_NUMB
  Logical : Logic  OutDataTypeStr=boolean
  GaCFM_AFECellVoltLineOpen_flg : Outport
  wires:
  LaCFM_AFECellVoltLineOpen_flg/1 -> Logical/1
  CFM_GaCFM_AFECellVoltLineOpen_flg/1 -> GaCFM_AFECellVoltLineOpen_flg/1  "GaCFM_AFECellVoltLineOpen_flg"
  Logical/1 -> CFM_GaCFM_AFECellVoltLineOpen_flg/1
  GaISP_AFEComLost_numb/1 -> Comparison4/1
  Comparison4/1 -> Logical/2
  Constant2/1 -> Comparison4/2

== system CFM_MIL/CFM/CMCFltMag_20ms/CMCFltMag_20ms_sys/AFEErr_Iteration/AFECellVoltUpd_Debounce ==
  LaCFM_AFECellVoltUpdErr_flg : Inport
  GaISP_AFEComLost_numb : Inport  Port=2
  CFM_GaCFM_AFECellVoltUpdErr_flg : AIWAYS_Powertrain_BMS_lib/Signals/OverWrite  OverWrite_Value=CaCFM_AFECellVoltUpdErrOvr_flg  OverWrite_flag=CbCFM_AFECellVoltUpdErrOvrSwt_flg
  Comparison4 : RelationalOperator  Operator===  OutDataTypeStr=boolean
  Constant3 : Constant  Value=CFM_CONST0_NUMB
  Logical : Logic  OutDataTypeStr=boolean
  GaCFM_AFECellVoltUpdErr_flg : Outport
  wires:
  Logical/1 -> CFM_GaCFM_AFECellVoltUpdErr_flg/1
  CFM_GaCFM_AFECellVoltUpdErr_flg/1 -> GaCFM_AFECellVoltUpdErr_flg/1  "GaCFM_AFECellVoltUpdErr_flg"
  Constant3/1 -> Comparison4/2
  GaISP_AFEComLost_numb/1 -> Comparison4/1
  Comparison4/1 -> Logical/2
  LaCFM_AFECellVoltUpdErr_flg/1 -> Logical/1

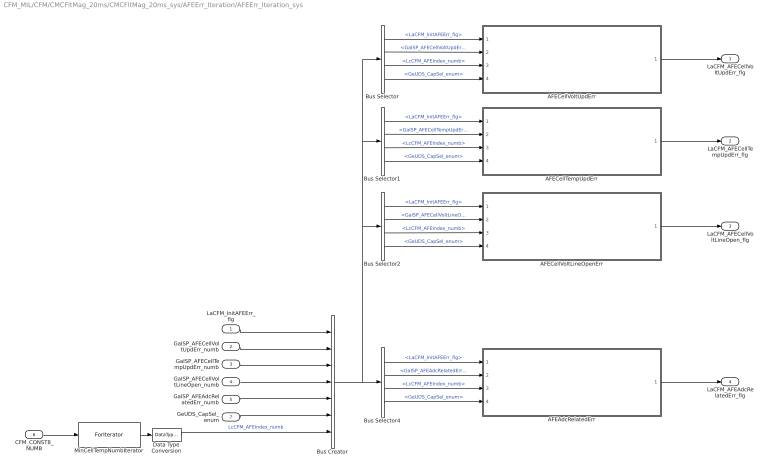
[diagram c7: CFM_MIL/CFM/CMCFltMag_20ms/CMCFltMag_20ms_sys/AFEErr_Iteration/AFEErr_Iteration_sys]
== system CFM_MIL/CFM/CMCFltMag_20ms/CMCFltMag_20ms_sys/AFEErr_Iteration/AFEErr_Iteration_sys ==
  LaCFM_InitAFEErr_flg : Inport
  GaISP_AFECellVoltUpdErr_numb : Inport  Port=2
  GaISP_AFECellTempUpdErr_numb : Inport  Port=3
  GaISP_AFECellVoltLineOpen_numb : Inport  Port=4
  GaISP_AFEAdcRelatedErr_numb : Inport  Port=5
  CFM_CONST8_NUMB : Inport  Port=6
  GeUDS_CapSel_enum : Inport  Port=7
  AFEAdcRelatedErr : Subsystem
  AFECellTempUpdErr : Subsystem
  AFECellVoltLineOpenErr : Subsystem
  AFECellVoltUpdErr : Subsystem
  Bus Creator : BusCreator  Inputs=7
  Bus Selector : BusSelector  OutputSignals=LaCFM_InitAFEErr_flg,GaISP_AFECellVoltUpdErr_numb,LcCFM_AFEIndex_numb,GeUDS_CapSel_enum
  Bus Selector1 : BusSelector  OutputSignals=LaCFM_InitAFEErr_flg,GaISP_AFECellTempUpdErr_numb,LcCFM_AFEIndex_numb,GeUDS_CapSel_enum
  Bus Selector2 : BusSelector  OutputSignals=LaCFM_InitAFEErr_flg,GaISP_AFECellVoltLineOpen_numb,LcCFM_AFEIndex_numb,GeUDS_CapSel_enum
  Bus Selector4 : BusSelector  OutputSignals=LaCFM_InitAFEErr_flg,GaISP_AFEAdcRelatedErr_numb,LcCFM_AFEIndex_numb,GeUDS_CapSel_enum
  Data Type Conversion : DataTypeConversion  OutDataTypeStr=uint8
  MinCellTempNumbIterator : ForIterator  ResetStates=reset  IterationSource=external  IterationVariableDataType=int8
  LaCFM_AFECellVoltUpdErr_flg : Outport
  LaCFM_AFECellTempUpdErr_flg : Outport  Port=2
  LaCFM_AFECellVoltLineOpen_flg : Outport  Port=3
  LaCFM_AFEAdcRelatedErr_flg : Outport  Port=4
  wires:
  MinCellTempNumbIterator/1 -> Data Type Conversion/1
  CFM_CONST8_NUMB/1 -> MinCellTempNumbIterator/1
  LaCFM_InitAFEErr_flg/1 -> Bus Creator/1
  GaISP_AFECellVoltUpdErr_numb/1 -> Bus Creator/2
  Data Type Conversion/1 -> Bus Creator/7  "LcCFM_AFEIndex_numb"
  Bus Creator/1 -> Bus Selector/1, Bus Selector1/1, Bus Selector2/1, Bus Selector4/1
  Bus Selector/1 -> AFECellVoltUpdErr/1(LaCFM_InitAFEErr_flg)  "<LaCFM_InitAFEErr_flg>"
  Bus Selector/2 -> AFECellVoltUpdErr/2(GaISP_AFECellVoltUpdErr_numb)  "<GaISP_AFECellVoltUpdErr_numb>"
  Bus Selector/3 -> AFECellVoltUpdErr/3(LcCFM_AFEIndex_numb)  "<LcCFM_AFEIndex_numb>"
  GaISP_AFECellTempUpdErr_numb/1 -> Bus Creator/3
  GaISP_AFECellVoltLineOpen_numb/1 -> Bus Creator/4
  GaISP_AFEAdcRelatedErr_numb/1 -> Bus Creator/5
  Bus Selector1/1 -> AFECellTempUpdErr/1(LaCFM_InitAFEErr_flg)  "<LaCFM_InitAFEErr_flg>"
  Bus Selector1/2 -> AFECellTempUpdErr/2(GaISP_AFECellTempUpdErr_numb)  "<GaISP_AFECellTempUpdErr_numb>"
  Bus Selector1/3 -> AFECellTempUpdErr/3(LcCFM_AFEIndex_numb)  "<LcCFM_AFEIndex_numb>"
  Bus Selector2/1 -> AFECellVoltLineOpenErr/1(LaCFM_InitAFEErr_flg)  "<LaCFM_InitAFEErr_flg>"
  Bus Selector2/2 -> AFECellVoltLineOpenErr/2(GaISP_AFECellVoltLineOpen_numb)  "<GaISP_AFECellVoltLineOpen_numb>"
  Bus Selector2/3 -> AFECellVoltLineOpenErr/3(LcCFM_AFEIndex_numb)  "<LcCFM_AFEIndex_numb>"
  Bus Selector4/1 -> AFEAdcRelatedErr/1(LaCFM_InitAFEErr_flg)  "<LaCFM_InitAFEErr_flg>"
  Bus Selector4/2 -> AFEAdcRelatedErr/2(GaISP_AFEAdcRelatedErr_numb)  "<GaISP_AFEAdcRelatedErr_numb>"
  Bus Selector4/3 -> AFEAdcRelatedErr/3(LcCFM_AFEIndex_numb)  "<LcCFM_AFEIndex_numb>"
  AFECellVoltLineOpenErr/1(LaCFM_AFECellVoltLineOpen_flg) -> LaCFM_AFECellVoltLineOpen_flg/1
  AFECellTempUpdErr/1(LaCFM_AFECellTempUpdErr_flg) -> LaCFM_AFECellTempUpdErr_flg/1
  AFECellVoltUpdErr/1(LaCFM_AFECellVoltUpdErr_flg) -> LaCFM_AFECellVoltUpdErr_flg/1
  AFEAdcRelatedErr/1(LaCFM_AFEAdcRelatedErr_flg) -> LaCFM_AFEAdcRelatedErr_flg/1
  GeUDS_CapSel_enum/1 -> Bus Creator/6
  Bus Selector/4 -> AFECellVoltUpdErr/4(GeUDS_CapSel_enum)  "<GeUDS_CapSel_enum>"
  Bus Selector1/4 -> AFECellTempUpdErr/4(GeUDS_CapSel_enum)  "<GeUDS_CapSel_enum>"
  Bus Selector2/4 -> AFECellVoltLineOpenErr/4(GeUDS_CapSel_enum)  "<GeUDS_CapSel_enum>"
  Bus Selector4/4 -> AFEAdcRelatedErr/4(GeUDS_CapSel_enum)  "<GeUDS_CapSel_enum>"

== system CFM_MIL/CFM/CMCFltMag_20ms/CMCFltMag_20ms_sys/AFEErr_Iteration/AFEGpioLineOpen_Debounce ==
  GaCDP_AFETempSampAbn_flg : Inport
  GaISP_AFEComLost_numb : Inport  Port=2
  CFM_GaCFM_AFEGpioLineOpen_flg : AIWAYS_Powertrain_BMS_lib/Signals/OverWrite  OverWrite_Value=CaCFM_AFEGpioLineOpenOvr_flg  OverWrite_flag=CbCFM_AFEGpioLineOpenOvrSwt_flg
  Comparison4 : RelationalOperator  Operator===  OutDataTypeStr=boolean
  Constant3 : Constant  Value=CFM_CONST0_NUMB
  Logical : Logic  OutDataTypeStr=boolean
  GaCFM_AFEGpioLineOpen_flg : Outport
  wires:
  Logical/1 -> CFM_GaCFM_AFEGpioLineOpen_flg/1
  CFM_GaCFM_AFEGpioLineOpen_flg/1 -> GaCFM_AFEGpioLineOpen_flg/1  "GaCFM_AFEGpioLineOpen_flg"
  GaISP_AFEComLost_numb/1 -> Comparison4/1
  Comparison4/1 -> Logical/2
  GaCDP_AFETempSampAbn_flg/1 -> Logical/1
  Constant3/1 -> Comparison4/2

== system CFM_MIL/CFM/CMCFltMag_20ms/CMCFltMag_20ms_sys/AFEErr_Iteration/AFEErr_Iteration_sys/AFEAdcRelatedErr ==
  LaCFM_InitAFEErr_flg : Inport
  GaISP_AFEAdcRelatedErr_numb : Inport  Port=2
  LcCFM_AFEIndex_numb : Inport  Port=3
  GeUDS_CapSel_enum : Inport  Port=4
  AFEAdcRelatedErr_sys : Subsystem
  Assignment : Assignment  DiagnosticForDimensions=Warning  IndexOptions=Index vector (port)  Indices=1  OutputSizes=1
  Constant2 : Constant  Value=CFM_CONST14_NUMB
  LaCFM_AFEAdcRelatedErr_flg : Outport
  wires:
  LaCFM_InitAFEErr_flg/1 -> Assignment/1
  GaISP_AFEAdcRelatedErr_numb/1 -> AFEAdcRelatedErr_sys/1(GaISP_AFEAdcRelatedErr_numb)
  LcCFM_AFEIndex_numb/1 -> AFEAdcRelatedErr_sys/2(LcCFM_AFEIndex_numb), Assignment/3
  Constant2/1 -> AFEAdcRelatedErr_sys/3(CFM_CONST14_NUMB)
  AFEAdcRelatedErr_sys/1(LbCFM_AFEAdcRelatedErr_flg) -> Assignment/2
  Assignment/1 -> LaCFM_AFEAdcRelatedErr_flg/1  "LaCFM_AFEAdcRelatedErr_flg"
  GeUDS_CapSel_enum/1 -> AFEAdcRelatedErr_sys/4(GeUDS_CapSel_enum)

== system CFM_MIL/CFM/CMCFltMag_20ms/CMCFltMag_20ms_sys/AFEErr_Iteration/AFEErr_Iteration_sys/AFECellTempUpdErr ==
  LaCFM_InitAFEErr_flg : Inport
  GaISP_AFECellTempUpdErr_numb : Inport  Port=2
  LcCFM_AFEIndex_numb : Inport  Port=3
  GeUDS_CapSel_enum : Inport  Port=4
  AFECellTempUpdErr_sys : Subsystem
  Assignment : Assignment  DiagnosticForDimensions=Warning  IndexOptions=Index vector (port)  Indices=1  OutputSizes=1
  Constant2 : Constant  Value=CFM_CONST6_NUMB
  LaCFM_AFECellTempUpdErr_flg : Outport
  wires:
  Assignment/1 -> LaCFM_AFECellTempUpdErr_flg/1  "LaCFM_AFECellTempUpdErr_flg"
  AFECellTempUpdErr_sys/1(LbCFM_AFETempUpdErr_flg) -> Assignment/2
  Constant2/1 -> AFECellTempUpdErr_sys/3(CFM_CONST6_NUMB)
  LcCFM_AFEIndex_numb/1 -> Assignment/3, AFECellTempUpdErr_sys/2(LcCFM_AFEIndex_numb)
  GaISP_AFECellTempUpdErr_numb/1 -> AFECellTempUpdErr_sys/1(GaISP_AFECellTempUpdErr_numb)
  LaCFM_InitAFEErr_flg/1 -> Assignment/1
  GeUDS_CapSel_enum/1 -> AFECellTempUpdErr_sys/4(GeUDS_CapSel_enum)

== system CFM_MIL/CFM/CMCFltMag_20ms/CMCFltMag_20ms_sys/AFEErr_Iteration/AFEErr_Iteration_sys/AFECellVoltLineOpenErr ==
  LaCFM_InitAFEErr_flg : Inport
  GaISP_AFECellVoltLineOpen_numb : Inport  Port=2
  LcCFM_AFEIndex_numb : Inport  Port=3
  GeUDS_CapSel_enum : Inport  Port=4
  AFECellVoltLineOpenErr_sys : Subsystem
  Assignment : Assignment  DiagnosticForDimensions=Warning  IndexOptions=Index vector (port)  Indices=1  OutputSizes=1
  Constant2 : Constant  Value=CFM_CONST14_NUMB
  LaCFM_AFECellVoltLineOpen_flg : Outport
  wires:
  Assignment/1 -> LaCFM_AFECellVoltLineOpen_flg/1  "LaCFM_AFECellVoltLineOpen_flg"
  AFECellVoltLineOpenErr_sys/1(LbCFM_AFECellVoltLineOpenErr_flg) -> Assignment/2
  Constant2/1 -> AFECellVoltLineOpenErr_sys/3(CFM_CONST14_NUMB)
  LcCFM_AFEIndex_numb/1 -> Assignment/3, AFECellVoltLineOpenErr_sys/2(LcCFM_AFEIndex_numb)
  GaISP_AFECellVoltLineOpen_numb/1 -> AFECellVoltLineOpenErr_sys/1(GaISP_AFECellVoltLineOpen_numb)
  LaCFM_InitAFEErr_flg/1 -> Assignment/1
  GeUDS_CapSel_enum/1 -> AFECellVoltLineOpenErr_sys/4(GeUDS_CapSel_enum)

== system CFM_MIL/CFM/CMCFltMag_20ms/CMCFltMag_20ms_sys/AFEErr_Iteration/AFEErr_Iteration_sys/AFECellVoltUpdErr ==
  LaCFM_InitAFEErr_flg : Inport
  GaISP_AFECellVoltUpdErr_numb : Inport  Port=2
  LcCFM_AFEIndex_numb : Inport  Port=3
  GeUDS_CapSel_enum : Inport  Port=4
  AFECellVoltUpdErr_sys : Subsystem
  Assignment : Assignment  DiagnosticForDimensions=Warning  IndexOptions=Index vector (port)  Indices=1  OutputSizes=1
  Constant2 : Constant  Value=CFM_CONST14_NUMB
  LaCFM_AFECellVoltUpdErr_flg : Outport
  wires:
  LaCFM_InitAFEErr_flg/1 -> Assignment/1
  GaISP_AFECellVoltUpdErr_numb/1 -> AFECellVoltUpdErr_sys/1(GaISP_AFECellVoltUpdErr_numb)
  LcCFM_AFEIndex_numb/1 -> AFECellVoltUpdErr_sys/2(LcCFM_AFEIndex_numb), Assignment/3
  Constant2/1 -> AFECellVoltUpdErr_sys/3(CFM_CONST14_NUMB)
  AFECellVoltUpdErr_sys/1(LbCFM_AFECellVoltUpdErr_flg) -> Assignment/2
  Assignment/1 -> LaCFM_AFECellVoltUpdErr_flg/1  "LaCFM_AFECellVoltUpdErr_flg"
  GeUDS_CapSel_enum/1 -> AFECellVoltUpdErr_sys/4(GeUDS_CapSel_enum)

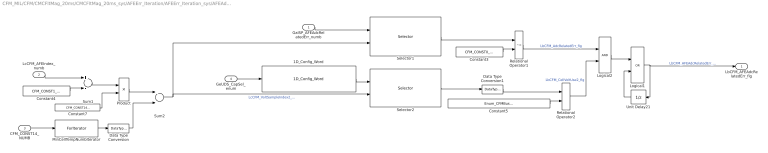
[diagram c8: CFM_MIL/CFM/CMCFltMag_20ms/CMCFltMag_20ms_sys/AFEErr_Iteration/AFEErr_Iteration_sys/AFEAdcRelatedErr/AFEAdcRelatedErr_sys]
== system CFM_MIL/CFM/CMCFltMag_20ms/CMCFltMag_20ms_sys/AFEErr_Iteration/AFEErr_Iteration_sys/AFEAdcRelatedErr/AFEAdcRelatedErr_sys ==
  GaISP_AFEAdcRelatedErr_numb : Inport
  LcCFM_AFEIndex_numb : Inport  Port=2
  CFM_CONST14_NUMB : Inport  Port=3
  GeUDS_CapSel_enum : Inport  Port=4
  1D_Config_Word : AIWAYS_Powertrain_BMS_lib/Signals/1D_Config_Word  Default_CalPar_Name=CaCFM_CATL177BusBarCell_enum  CATL153Ah_CalPar_Name=CaCFM_CATL177BusBarCell_enum  CATL180Ah_CalPar_Name=CaCFM_CATL177BusBarCell_enum  CATL177Ah_CalPar_Name=CaCFM_CATL177BusBarCell_enum  CATL203Ah_CalPar_Name=CaCFM_CATL203BusBarCell_enum  CATL51Ah_CalPar_Name=CaCFM_CATL177BusBarCell_enum  CATL132Ah_CalPar_Name=CaCFM_CATL177BusBarCell_enum  XWD75Ah_CalPar_Name=CaCFM_XWD75BusBarCell_enum  TFE177Ah_CalPar_Name=CaCFM_TFE177BusBarCell_enum  CATLCTP248Ah_CalPar_Name=CaCFM_CATL177BusBarCell_enum
  Constant3 : Constant  Value=CFM_CONST0_NUMB
  Constant4 : Constant  Value=CFM_CONST1_NUMB
  Constant5 : Constant  Value=Enum_CFMBusBarCell.Enum_CFMBusBarCell_Cell
  Constant7 : Constant  Value=CFM_CONST14_NUMB
  Data Type Conversion : DataTypeConversion  OutDataTypeStr=uint16
  Data Type Conversion1 : DataTypeConversion
  Logical1 : Logic  Operator=OR  OutDataTypeStr=boolean
  Logical2 : Logic  OutDataTypeStr=boolean
  MinCellTempNumbIterator : ForIterator  ResetStates=reset  IterationSource=external  IterationVariableDataType=int8
  Product : Product  OutDataTypeStr=Inherit: Inherit via back propagation
  Relational Operator1 : RelationalOperator  Operator=~=  OutDataTypeStr=boolean
  Relational Operator2 : RelationalOperator  Operator===  OutDataTypeStr=boolean
  Selector1 : Selector  IndexOptions=Index vector (port)  Indices=[1 3]  OutputSizes=1
  Selector2 : Selector  IndexOptions=Index vector (port)  Indices=[1 3]  OutputSizes=1
  Sum1 : Sum  Inputs=+-  OutDataTypeStr=Inherit: Inherit via back propagation  RndMeth=Zero
  Sum2 : Sum  OutDataTypeStr=Inherit: Inherit via back propagation  RndMeth=Zero
  Unit Delay21 : UnitDelay  InitialCondition=ASWTYPE_FALSE  SampleTime=-1  StateName=StateName
  LbCFM_AFEAdcRelatedErr_flg : Outport
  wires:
  Relational Operator2/1 -> Logical2/2  "LbCFM_CellVoltUse2_flg"
  Relational Operator1/1 -> Logical2/1  "LbCFM_AdcRelatedErr_flg"
  1D_Config_Word/1 -> Selector2/1
  GaISP_AFEAdcRelatedErr_numb/1 -> Selector1/1
  Constant3/1 -> Relational Operator1/2
  Selector2/1 -> Data Type Conversion1/1
  Constant5/1 -> Relational Operator2/2
  Selector1/1 -> Relational Operator1/1
  CFM_CONST14_NUMB/1 -> MinCellTempNumbIterator/1
  MinCellTempNumbIterator/1 -> Data Type Conversion/1
  Constant4/1 -> Sum1/2
  LcCFM_AFEIndex_numb/1 -> Sum1/1
  Sum1/1 -> Product/1
  Constant7/1 -> Product/2
  Product/1 -> Sum2/1
  Data Type Conversion/1 -> Sum2/2
  Sum2/1 -> Selector2/2, Selector1/2  "LcCFM_VoltSampleIndex2_numb"
  Logical2/1 -> Logical1/1
  Unit Delay21/1 -> Logical1/2
  Logical1/1 -> LbCFM_AFEAdcRelatedErr_flg/1, Unit Delay21/1  "LbCFM_AFEAdcRelatedErr_flg"
  Data Type Conversion1/1 -> Relational Operator2/1
  GeUDS_CapSel_enum/1 -> 1D_Config_Word/1

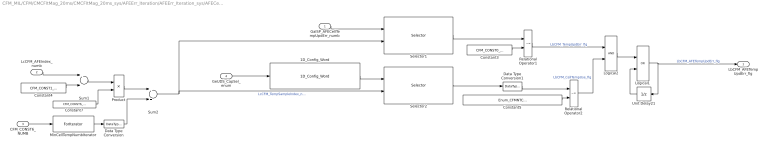
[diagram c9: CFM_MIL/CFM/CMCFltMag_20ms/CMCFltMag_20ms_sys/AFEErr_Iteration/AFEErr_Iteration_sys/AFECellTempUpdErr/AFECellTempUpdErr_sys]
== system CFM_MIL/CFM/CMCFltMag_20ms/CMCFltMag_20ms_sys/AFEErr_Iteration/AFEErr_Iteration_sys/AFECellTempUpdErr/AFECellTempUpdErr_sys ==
  GaISP_AFECellTempUpdErr_numb : Inport
  LcCFM_AFEIndex_numb : Inport  Port=2
  CFM_CONST6_NUMB : Inport  Port=3
  GeUDS_CapSel_enum : Inport  Port=4
  1D_Config_Word : AIWAYS_Powertrain_BMS_lib/Signals/1D_Config_Word  Default_CalPar_Name=CaCFM_CATL177NTCTemp_enum  CATL153Ah_CalPar_Name=CaCFM_CATL177NTCTemp_enum  CATL180Ah_CalPar_Name=CaCFM_CATL177NTCTemp_enum  CATL177Ah_CalPar_Name=CaCFM_CATL177NTCTemp_enum  CATL203Ah_CalPar_Name=CaCFM_CATL203NTCTemp_enum  CATL51Ah_CalPar_Name=CaCFM_CATL177NTCTemp_enum  CATL132Ah_CalPar_Name=CaCFM_CATL177NTCTemp_enum  XWD75Ah_CalPar_Name=CaCFM_XWD75NTCTemp_enum  TFE177Ah_CalPar_Name=CaCFM_TFE177NTCTemp_enum  CATLCTP248Ah_CalPar_Name=CaCFM_CATL177NTCTemp_enum
  Constant3 : Constant  Value=CFM_CONST0_NUMB
  Constant4 : Constant  Value=CFM_CONST1_NUMB
  Constant5 : Constant  Value=Enum_CFMNTCTemp.Enum_CFMNTCTemp_NoUse
  Constant7 : Constant  Value=CFM_CONST6_NUMB
  Data Type Conversion : DataTypeConversion  OutDataTypeStr=uint16
  Data Type Conversion1 : DataTypeConversion
  Logical1 : Logic  Operator=OR  OutDataTypeStr=boolean
  Logical2 : Logic  OutDataTypeStr=boolean
  MinCellTempNumbIterator : ForIterator  ResetStates=reset  IterationSource=external  IterationVariableDataType=int8
  Product : Product  OutDataTypeStr=Inherit: Inherit via back propagation
  Relational Operator1 : RelationalOperator  Operator=~=  OutDataTypeStr=boolean
  Relational Operator2 : RelationalOperator  Operator=~=  OutDataTypeStr=boolean
  Selector1 : Selector  IndexOptions=Index vector (port)  Indices=[1 3]  OutputSizes=1
  Selector2 : Selector  IndexOptions=Index vector (port)  Indices=[1 3]  OutputSizes=1
  Sum1 : Sum  Inputs=+-  OutDataTypeStr=Inherit: Inherit via back propagation  RndMeth=Zero
  Sum2 : Sum  OutDataTypeStr=Inherit: Inherit via back propagation  RndMeth=Zero
  Unit Delay21 : UnitDelay  InitialCondition=ASWTYPE_FALSE  SampleTime=-1  StateName=StateName
  LbCFM_AFETempUpdErr_flg : Outport
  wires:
  Logical1/1 -> Unit Delay21/1, LbCFM_AFETempUpdErr_flg/1  "LbCFM_AFETempUpdErr_flg"
  Unit Delay21/1 -> Logical1/2
  Logical2/1 -> Logical1/1
  Sum2/1 -> Selector2/2, Selector1/2  "LcCFM_TempSampleIndex_numb"
  Data Type Conversion/1 -> Sum2/2
  Product/1 -> Sum2/1
  Constant7/1 -> Product/2
  Sum1/1 -> Product/1
  LcCFM_AFEIndex_numb/1 -> Sum1/1
  Constant4/1 -> Sum1/2
  MinCellTempNumbIterator/1 -> Data Type Conversion/1
  CFM_CONST6_NUMB/1 -> MinCellTempNumbIterator/1
  Selector1/1 -> Relational Operator1/1
  Constant5/1 -> Relational Operator2/2
  Selector2/1 -> Data Type Conversion1/1
  Constant3/1 -> Relational Operator1/2
  GaISP_AFECellTempUpdErr_numb/1 -> Selector1/1
  1D_Config_Word/1 -> Selector2/1
  Relational Operator1/1 -> Logical2/1  "LbCFM_TempUpdErr_flg"
  Relational Operator2/1 -> Logical2/2  "LbCFM_CellTempUse_flg"
  Data Type Conversion1/1 -> Relational Operator2/1
  GeUDS_CapSel_enum/1 -> 1D_Config_Word/1

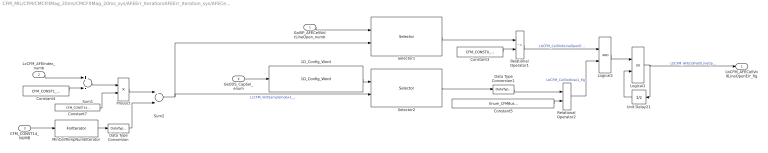
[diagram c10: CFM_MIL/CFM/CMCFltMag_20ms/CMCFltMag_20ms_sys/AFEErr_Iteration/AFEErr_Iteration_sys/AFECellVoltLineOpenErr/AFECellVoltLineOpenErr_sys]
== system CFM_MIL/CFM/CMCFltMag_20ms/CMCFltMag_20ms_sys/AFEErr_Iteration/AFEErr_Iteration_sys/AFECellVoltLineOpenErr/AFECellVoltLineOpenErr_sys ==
  GaISP_AFECellVoltLineOpen_numb : Inport
  LcCFM_AFEIndex_numb : Inport  Port=2
  CFM_CONST14_NUMB : Inport  Port=3
  GeUDS_CapSel_enum : Inport  Port=4
  1D_Config_Word : AIWAYS_Powertrain_BMS_lib/Signals/1D_Config_Word  Default_CalPar_Name=CaCFM_CATL177BusBarCell_enum  CATL153Ah_CalPar_Name=CaCFM_CATL177BusBarCell_enum  CATL180Ah_CalPar_Name=CaCFM_CATL177BusBarCell_enum  CATL177Ah_CalPar_Name=CaCFM_CATL177BusBarCell_enum  CATL203Ah_CalPar_Name=CaCFM_CATL203BusBarCell_enum  CATL51Ah_CalPar_Name=CaCFM_CATL177BusBarCell_enum  CATL132Ah_CalPar_Name=CaCFM_CATL177BusBarCell_enum  XWD75Ah_CalPar_Name=CaCFM_XWD75BusBarCell_enum  TFE177Ah_CalPar_Name=CaCFM_TFE177BusBarCell_enum  CATLCTP248Ah_CalPar_Name=CaCFM_CATL177BusBarCell_enum
  Constant3 : Constant  Value=CFM_CONST0_NUMB
  Constant4 : Constant  Value=CFM_CONST1_NUMB
  Constant5 : Constant  Value=Enum_CFMBusBarCell.Enum_CFMBusBarCell_Cell
  Constant7 : Constant  Value=CFM_CONST14_NUMB
  Data Type Conversion : DataTypeConversion  OutDataTypeStr=uint16
  Data Type Conversion1 : DataTypeConversion
  Logical1 : Logic  Operator=OR  OutDataTypeStr=boolean
  Logical2 : Logic  OutDataTypeStr=boolean
  MinCellTempNumbIterator : ForIterator  ResetStates=reset  IterationSource=external  IterationVariableDataType=int8
  Product : Product  OutDataTypeStr=Inherit: Inherit via back propagation
  Relational Operator1 : RelationalOperator  Operator=~=  OutDataTypeStr=boolean
  Relational Operator2 : RelationalOperator  Operator===  OutDataTypeStr=boolean
  Selector1 : Selector  IndexOptions=Index vector (port)  Indices=[1 3]  OutputSizes=1
  Selector2 : Selector  IndexOptions=Index vector (port)  Indices=[1 3]  OutputSizes=1
  Sum1 : Sum  Inputs=+-  OutDataTypeStr=Inherit: Inherit via back propagation  RndMeth=Zero
  Sum2 : Sum  OutDataTypeStr=Inherit: Inherit via back propagation  RndMeth=Zero
  Unit Delay21 : UnitDelay  InitialCondition=ASWTYPE_FALSE  SampleTime=-1  StateName=StateName
  LbCFM_AFECellVoltLineOpenErr_flg : Outport
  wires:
  Logical1/1 -> Unit Delay21/1, LbCFM_AFECellVoltLineOpenErr_flg/1  "LbCFM_AFECellVoltLineOpenErr_flg"
  Unit Delay21/1 -> Logical1/2
  Logical2/1 -> Logical1/1
  Sum2/1 -> Selector2/2, Selector1/2  "LcCFM_VoltSampleIndex1_numb"
  Data Type Conversion/1 -> Sum2/2
  Product/1 -> Sum2/1
  Constant7/1 -> Product/2
  Sum1/1 -> Product/1
  LcCFM_AFEIndex_numb/1 -> Sum1/1
  Constant4/1 -> Sum1/2
  MinCellTempNumbIterator/1 -> Data Type Conversion/1
  CFM_CONST14_NUMB/1 -> MinCellTempNumbIterator/1
  Selector1/1 -> Relational Operator1/1
  Constant5/1 -> Relational Operator2/2
  Selector2/1 -> Data Type Conversion1/1
  Constant3/1 -> Relational Operator1/2
  GaISP_AFECellVoltLineOpen_numb/1 -> Selector1/1
  1D_Config_Word/1 -> Selector2/1
  Relational Operator1/1 -> Logical2/1  "LbCFM_CellVoltLineOpenErr_flg"
  Relational Operator2/1 -> Logical2/2  "LbCFM_CellVoltUse1_flg"
  Data Type Conversion1/1 -> Relational Operator2/1
  GeUDS_CapSel_enum/1 -> 1D_Config_Word/1

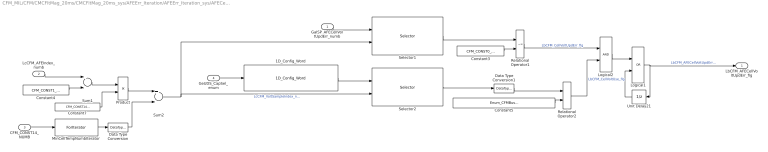
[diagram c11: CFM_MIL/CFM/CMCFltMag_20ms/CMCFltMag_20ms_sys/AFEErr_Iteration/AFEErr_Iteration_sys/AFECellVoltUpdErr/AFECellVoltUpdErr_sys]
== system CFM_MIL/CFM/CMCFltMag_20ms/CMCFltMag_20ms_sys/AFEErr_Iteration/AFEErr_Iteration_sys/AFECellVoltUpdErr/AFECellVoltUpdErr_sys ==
  GaISP_AFECellVoltUpdErr_numb : Inport
  LcCFM_AFEIndex_numb : Inport  Port=2
  CFM_CONST14_NUMB : Inport  Port=3
  GeUDS_CapSel_enum : Inport  Port=4
  1D_Config_Word : AIWAYS_Powertrain_BMS_lib/Signals/1D_Config_Word  Default_CalPar_Name=CaCFM_CATL177BusBarCell_enum  CATL153Ah_CalPar_Name=CaCFM_CATL177BusBarCell_enum  CATL180Ah_CalPar_Name=CaCFM_CATL177BusBarCell_enum  CATL177Ah_CalPar_Name=CaCFM_CATL177BusBarCell_enum  CATL203Ah_CalPar_Name=CaCFM_CATL203BusBarCell_enum  CATL51Ah_CalPar_Name=CaCFM_CATL177BusBarCell_enum  CATL132Ah_CalPar_Name=CaCFM_CATL177BusBarCell_enum  XWD75Ah_CalPar_Name=CaCFM_XWD75BusBarCell_enum  TFE177Ah_CalPar_Name=CaCFM_TFE177BusBarCell_enum  CATLCTP248Ah_CalPar_Name=CaCFM_CATL177BusBarCell_enum
  Constant3 : Constant  Value=CFM_CONST0_NUMB
  Constant4 : Constant  Value=CFM_CONST1_NUMB
  Constant5 : Constant  Value=Enum_CFMBusBarCell.Enum_CFMBusBarCell_Cell
  Constant7 : Constant  Value=CFM_CONST14_NUMB
  Data Type Conversion : DataTypeConversion  OutDataTypeStr=uint16
  Data Type Conversion1 : DataTypeConversion
  Logical1 : Logic  Operator=OR  OutDataTypeStr=boolean
  Logical2 : Logic  OutDataTypeStr=boolean
  MinCellTempNumbIterator : ForIterator  ResetStates=reset  IterationSource=external  IterationVariableDataType=int8
  Product : Product  OutDataTypeStr=Inherit: Inherit via back propagation
  Relational Operator1 : RelationalOperator  Operator=~=  OutDataTypeStr=boolean
  Relational Operator2 : RelationalOperator  Operator===  OutDataTypeStr=boolean
  Selector1 : Selector  IndexOptions=Index vector (port)  Indices=[1 3]  OutputSizes=1
  Selector2 : Selector  IndexOptions=Index vector (port)  Indices=[1 3]  OutputSizes=1
  Sum1 : Sum  Inputs=+-  OutDataTypeStr=Inherit: Inherit via back propagation  RndMeth=Zero
  Sum2 : Sum  OutDataTypeStr=Inherit: Inherit via back propagation  RndMeth=Zero
  Unit Delay21 : UnitDelay  InitialCondition=ASWTYPE_FALSE  SampleTime=-1  StateName=StateName
  LbCFM_AFECellVoltUpdErr_flg : Outport
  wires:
  Relational Operator2/1 -> Logical2/2  "LbCFM_CellVoltUse_flg"
  Relational Operator1/1 -> Logical2/1  "LbCFM_CellVoltUpdErr_flg"
  1D_Config_Word/1 -> Selector2/1
  GaISP_AFECellVoltUpdErr_numb/1 -> Selector1/1
  Constant3/1 -> Relational Operator1/2
  Selector2/1 -> Data Type Conversion1/1
  Constant5/1 -> Relational Operator2/2
  Selector1/1 -> Relational Operator1/1
  CFM_CONST14_NUMB/1 -> MinCellTempNumbIterator/1
  MinCellTempNumbIterator/1 -> Data Type Conversion/1
  Constant4/1 -> Sum1/2
  LcCFM_AFEIndex_numb/1 -> Sum1/1
  Sum1/1 -> Product/1
  Constant7/1 -> Product/2
  Product/1 -> Sum2/1
  Data Type Conversion/1 -> Sum2/2
  Sum2/1 -> Selector2/2, Selector1/2  "LcCFM_VoltSampleIndex_numb"
  Logical2/1 -> Logical1/1
  Unit Delay21/1 -> Logical1/2
  Logical1/1 -> LbCFM_AFECellVoltUpdErr_flg/1, Unit Delay21/1  "LbCFM_AFECellVoltUpdErr_flg"
  Data Type Conversion1/1 -> Relational Operator2/1
  GeUDS_CapSel_enum/1 -> 1D_Config_Word/1

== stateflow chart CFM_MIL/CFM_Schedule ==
  (default) -> (junction 13)
  (junction 13) -> (junction 150) : { TimeCounter20ms ++; }
  (junction 150) -> (junction 422) : [TimeCounter20ms >= Const20ms]
  (junction 150) -> (junction 424)
  (junction 422) -> (junction 424) : { CFM_CMCFltMag_20ms; TimeCounter20ms = 0; }
  data: TimeCounter20ms local uint8; Const20ms constant uint8 =2
  events: output FUNCTION_CALL_EVENT
